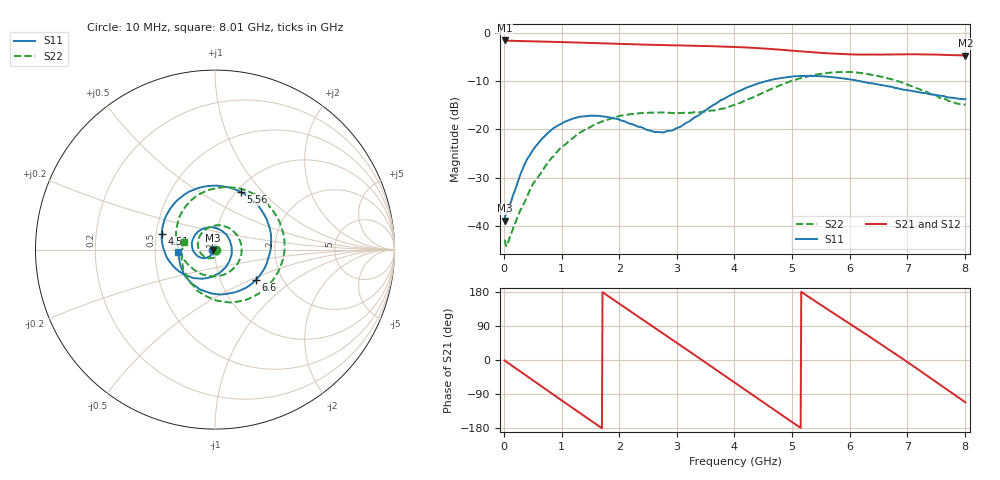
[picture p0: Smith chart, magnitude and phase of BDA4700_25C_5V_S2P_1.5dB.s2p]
!Agilent Technologies,E5071B,MY42404982,A.09.10
!Date: Mon Oct 20 13:26:40 2025
!Data & Calibration Information:
!Freq	S11:SOLT2(ON)	S21:SOLT2(ON)	S12:SOLT2(ON)	S22:SOLT2(ON)
# Hz S RI R 50
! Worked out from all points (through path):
!   801 points, 10 MHz to 8.01 GHz, reference 50 ohm
!   highest |S21| = -1.62 dB at 10 MHz (marker M1); lowest = -4.7 dB at 8.01 GHz (marker M2)
!   group delay of S21, straight-line fit = 287 ps
!   lowest |S11| = -38.9 dB at 10 MHz (marker M3), VSWR 1.02, Z = 48.9 - j0.208 ohm
!   |S11| at or under -10 dB: start of sweep to 4.569 GHz; 6.153 GHz to end of sweep
!   |S22| runs from -44.2 to -8.1 dB; largest |S21 - S12| = 0.0061
!   S11 on the Smith chart (normalised r, x): 10 MHz: 0.98, -0.00; 4.51 GHz: 0.53, +0.10; 5.56 GHz: 1.05, +0.77; 6.6 GHz: 1.46, -0.54; 8.01 GHz: 0.66, -0.02
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1e7  -0.0111 -0.00213  0.8294 -0.0178  0.8292 -0.0186  0.00712 -0.00108
3.7e8  -0.0271 -0.0358  0.6274 -0.5222  0.6268 -0.5226  0.0151 -0.0101
7.2e8  -0.0731 -0.0465  0.1826 -0.7853  0.1826 -0.7856  -0.00109 -0.0417
1.02e9  -0.1151 -0.0169  -0.2541 -0.7557  -0.2543 -0.7561  -0.0493 -0.0448
1.35e9  -0.1269 0.0466  -0.6311 -0.4701  -0.6314 -0.4703  -0.0939 0.0109
1.64e9  -0.0941 0.1005  -0.7721 -0.0845  -0.7723 -0.0848  -0.0786 0.0857
1.92e9  -0.0351 0.1242  -0.7058 0.2994  -0.7064 0.2996  -0.00755 0.1326
2.32e9  0.0515 0.0932  -0.3254 0.6797  -0.325 0.6805  0.1134 0.0919
2.68e9  0.092 0.0186  0.1502 0.7301  0.1503 0.73  0.1469 -0.0254
3.36e9  0.012 -0.1367  0.7232 0.0995  0.7237 0.0985  -0.0133 -0.1489
3.67e9  -0.0868 -0.1612  0.6564 -0.2998  0.6564 -0.3017  -0.0984 -0.1227
4.01e9  -0.2071 -0.1159  0.3526 -0.6174  0.3534 -0.6172  -0.169 -0.0607
4.51e9  -0.2971 0.0882  -0.2666 -0.6311  -0.2667 -0.6316  -0.2166 0.1058
4.93e9  -0.1996 0.2835  -0.6025 -0.2604  -0.6025 -0.2626  -0.1281 0.279
5.35e9  0.0239 0.3551  -0.5915 0.2088  -0.5924 0.2076  0.1 0.3452
5.56e9  0.1432 0.3215  -0.467 0.399  -0.4677 0.3991  0.2256 0.3049
6.07e9  0.3104 0.092  0.0138 0.5935  0.0136 0.5959  0.3873 0.0311
6.6e9  0.2263 -0.171  0.4819 0.3474  0.4826 0.3458  0.2408 -0.2466
6.68e9  0.1945 -0.1986  0.5258 0.2753  0.527 0.2745  0.1992 -0.2684
7.23e9  -0.0495 -0.2344  0.5212 -0.2912  0.5207 -0.2929  -0.0694 -0.2473
7.63e9  -0.1716 -0.1386  0.1872 -0.5583  0.1862 -0.5595  -0.1769 -0.1112
8.01e9  -0.2044 -0.016  -0.2143 -0.538  -0.2139 -0.5384  -0.1751 0.0397
